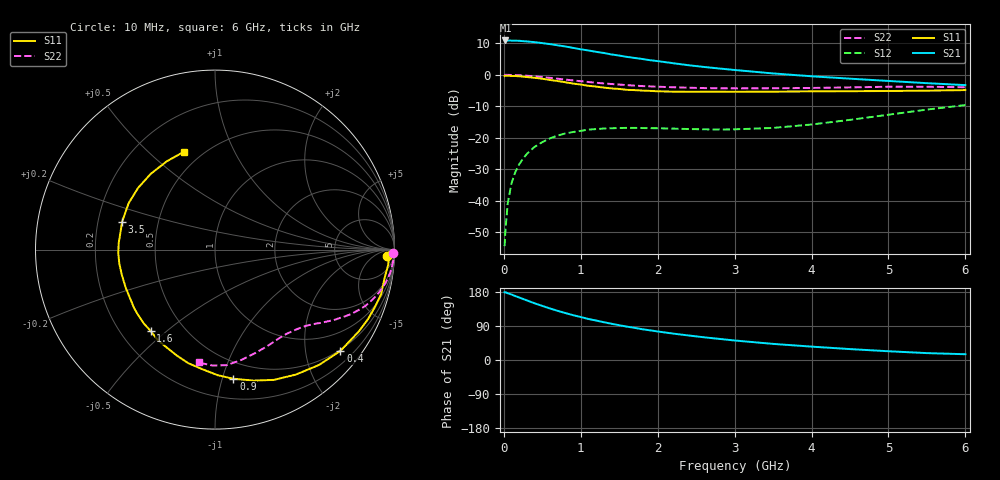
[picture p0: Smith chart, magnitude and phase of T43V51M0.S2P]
! Infineon Technologies  Discrete & RF Semiconductors
! BFR182T
! Si NPN RF Bipolar Junction Transistor in SC75
! VCE = 3.5 V  IC = 1 mA
! Common Emitter S-Parameters:  October  1999
# GHz  S  MA  R  50
!  f  S11  S21  S12  S22
! GHz  MAG  ANG  MAG  ANG  MAG  ANG  MAG  ANG
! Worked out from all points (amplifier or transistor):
!   36 points, 10 MHz to 6 GHz, reference 50 ohm
!   highest |S21| = 10.9 dB at 20 MHz (marker M1)
!   |S21| within 3 dB of that: start of sweep to 1.052 GHz
!   unconditionally stable (mu >= 1): 2.392 GHz to 4.562 GHz
!   at 250 MHz: K = 0.08, MSG = 18.7 dB, |S12| = -26.6 dB
!   at 1.4 GHz: K = 0.58, MSG = 11.7 dB, |S12| = -17.0 dB
!   at 6 GHz: K = 0.83, MSG = 3.2 dB, |S12| = -9.6 dB
!   S11 on the Smith chart (normalised r, x): 10 MHz: 28, -22; 400 MHz: 0.47, -2.76; 900 MHz: 0.36, -1.09; 1.6 GHz: 0.32, -0.44; 3.5 GHz: 0.30, +0.13; 6 GHz: 0.40, +0.65
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0.01  0.9561 -2.0  3.484 178.7  0.0019 95.9  0.9917 -1.1
0.02  0.9728 -0.7  3.514 178.9  0.0033 103.6  0.9999 -0.7
0.05  0.9688 -5.0  3.509 176.2  0.009 92.2  0.9972 -2.0
0.1  0.9582 -9.5  3.493 172.8  0.0191 85.6  0.9943 -3.8
0.15  0.958 -15.1  3.484 168.7  0.0288 80.9  0.9898 -5.7
0.25  0.9363 -24.4  3.428 161.1  0.0466 76.4  0.9763 -9.4
0.4  0.8981 -38.9  3.304 149.6  0.0719 67.3  0.9451 -14.6
0.5  0.8657 -47.9  3.191 142.7  0.0853 62.6  0.9209 -17.6
0.6  0.8293 -57.1  3.074 135.9  0.0978 57.9  0.895 -20.5
0.7  0.7969 -65.6  2.941 129.7  0.1087 53.8  0.8671 -22.9
0.8  0.7613 -73.5  2.817 123.9  0.1172 50.0  0.8406 -25.2
0.9  0.7268 -81.9  2.68 118.3  0.1235 46.6  0.814 -27.2
1.1  0.6696 -96.2  2.438 108.2  0.1349 41.1  0.7694 -30.7
1.4  0.6082 -116.3  2.106 95.6  0.1416 34.5  0.7148 -34.9
1.6  0.5776 -128.4  1.928 88.0  0.1436 32.1  0.686 -37.3
1.8  0.5626 -139.5  1.785 81.2  0.1429 30.5  0.6626 -39.8
2.2  0.5408 -156.9  1.53 69.7  0.1399 30.1  0.6353 -44.4
2.8  0.5392 -177.8  1.26 55.7  0.1355 34.5  0.6111 -52.4
3.5  0.5402 163.2  1.052 42.5  0.1435 45.7  0.6119 -61.7
4.5  0.5494 141.2  0.869 28.8  0.1926 58.3  0.6317 -76.4
5.5  0.5604 118.6  0.737 18.2  0.2804 60.2  0.6462 -91.3
6  0.572 107.7  0.686 15.2  0.3313 57.6  0.6353 -98.3
